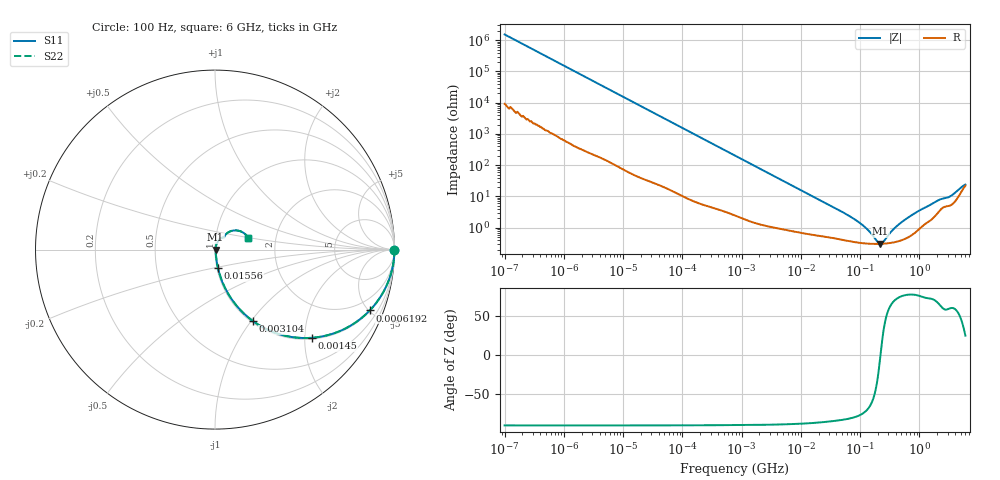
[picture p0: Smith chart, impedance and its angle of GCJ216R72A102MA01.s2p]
!Murata Part Number: GCJ216R72A102MA01
!These Parameters are Measured in Series Mode Connection
!Data Generated on Mar 13, 2026
!  o--ll--o
!Port1  Port2
!  o------o
!Operation Temp=25[degC], DC Bias Voltage=0[V]
!Freq. Start=100[Hz] Stop=6[GHz] 401[Steps]
# Hz S RI R 50
!Freq.(Hz) S11(Real) S11(Imag) S21(Real) S21(Imag) S12(Real) S12(Imag) S22(Real) S22(Imag)
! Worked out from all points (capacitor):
!   401 points, 100 Hz to 6 GHz, reference 50 ohm
!   read as one part in series: C = 1.04 nF near 109 Hz
!   lowest |Z| = 305 mohm at 218.4 MHz (marker M1)
!   series resonance near 221.3 MHz, so ESL is about 500 pH
!   S11 on the Smith chart (normalised r, x): 100 Hz: open; 619.2 kHz: 1.06, -5.07; 1.45 MHz: 1.03, -2.18; 3.104 MHz: 1.02, -1.02; 15.56 MHz: 1.01, -0.21; 6 GHz: 1.44, +0.20
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100  1 -6.56e-05  4e-07 6.56e-05  4e-07 6.56e-05  1 -6.56e-05
164  1 -0.000107  6e-07 0.000107  6e-07 0.000107  1 -0.000107
2008  1 -0.00131  7.1e-06 0.00131  7.1e-06 0.00131  1 -0.00131
40335  0.9992 -0.026  0.000832 0.026  0.000832 0.026  0.9992 -0.026
184852  0.9853 -0.1167  0.0147 0.1167  0.0147 0.1167  0.9853 -0.1167
619225  0.8625 -0.3387  0.1375 0.3387  0.1375 0.3387  0.8625 -0.3387
774597  0.8018 -0.3927  0.1982 0.3927  0.1982 0.3927  0.8018 -0.3927
1449809  0.5418 -0.4912  0.4582 0.4912  0.4582 0.4912  0.5418 -0.4912
3103719  0.2118 -0.3983  0.7882 0.3983  0.7882 0.3983  0.2118 -0.3983
6075234  0.0711 -0.2418  0.9289 0.2418  0.9289 0.2418  0.0711 -0.2418
1.555665e7  0.0163 -0.1012  0.9837 0.1012  0.9837 0.1012  0.0163 -0.1012
8.918374e7  0.0036 -0.0159  0.9964 0.0159  0.9964 0.0159  0.0036 -0.0159
1.275994e8  0.00318 -0.00895  0.9968 0.00895  0.9968 0.00895  0.00318 -0.00895
1.996653e8  0.00302 -0.0016  0.997 0.0016  0.997 0.0016  0.00302 -0.0016
2.183701e8  0.00303 -0.000207  0.997 0.000207  0.997 0.000207  0.00303 -0.000207
2.497637e8  0.00308 0.00189  0.9969 -0.00189  0.9969 -0.00189  0.00308 0.00189
3.124326e8  0.00324 0.00549  0.9968 -0.00549  0.9968 -0.00549  0.00324 0.00549
4.674818e8  0.00394 0.0129  0.9961 -0.0129  0.9961 -0.0129  0.00394 0.0129
8.366708e8  0.0075 0.0277  0.9925 -0.0277  0.9925 -0.0277  0.0075 0.0277
2.048624e9  0.033 0.0636  0.967 -0.0636  0.967 -0.0636  0.033 0.0636
3.505958e9  0.0588 0.083  0.9412 -0.083  0.9412 -0.083  0.0588 0.083
6e9  0.1849 0.0664  0.8151 -0.0664  0.8151 -0.0664  0.1849 0.0664
